FUNCTION "FC_PROG_L1" : VOID
TITLE =FC PROG OVEN LINE 1
{ S7_language := '9(1) Angielski (Stany Zjednoczone)  11.01.2022  09:45:15' }
VERSION : 0.1


VAR_TEMP
  DoorOK : BOOL ;
  ECooling_SP : REAL ;
END_VAR
BEGIN
NETWORK
TITLE =SET FULL PRODUCTION OR REDUCED PRODUCTION MODE
//THIS MODE WILL BE USE AFTER IN SETTING SETPOINTS FOR OVEN FANS (=15FAN01,
//=20FAN01)
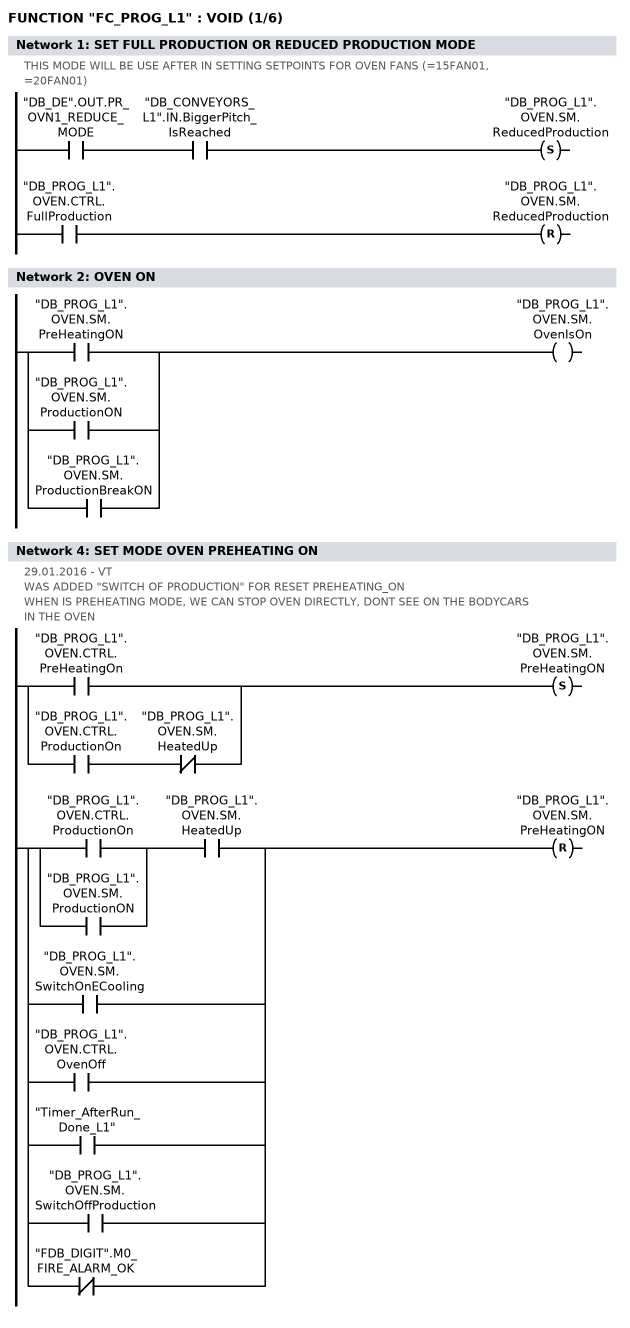
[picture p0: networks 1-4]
      U     "DB_DE".OUT.PR_OVN1_REDUCE_MODE;
      U     "DB_CONVEYORS_L1".IN.BiggerPitch_IsReached;
      S     "DB_PROG_L1".OVEN.SM.ReducedProduction;
      U     "DB_PROG_L1".OVEN.CTRL.FullProduction;
      R     "DB_PROG_L1".OVEN.SM.ReducedProduction;
      NOP   0;
NETWORK
TITLE =OVEN ON

      O     "DB_PROG_L1".OVEN.SM.PreHeatingON;
      O     "DB_PROG_L1".OVEN.SM.ProductionON;
      O     "DB_PROG_L1".OVEN.SM.ProductionBreakON;
      =     "DB_PROG_L1".OVEN.SM.OvenIsOn;
NETWORK
TITLE =SET MODE OF OVEN
//
//************************** SET MODE OF OVEN **********************************
//
NETWORK
TITLE =SET MODE OVEN PREHEATING ON
//29.01.2016 - VT
//WAS ADDED "SWITCH OF PRODUCTION" FOR RESET PREHEATING_ON
//WHEN IS PREHEATING MODE, WE CAN STOP OVEN DIRECTLY, DONT SEE ON THE BODYCARS
//IN THE OVEN
      U(    ;
      O     "DB_PROG_L1".OVEN.CTRL.PreHeatingOn;
      O     ;
      U     "DB_PROG_L1".OVEN.CTRL.ProductionOn;
      UN    "DB_PROG_L1".OVEN.SM.HeatedUp;
      )     ;
      S     "DB_PROG_L1".OVEN.SM.PreHeatingON;
      U(    ;
      U(    ;
      O     "DB_PROG_L1".OVEN.CTRL.ProductionOn;
      O     "DB_PROG_L1".OVEN.SM.ProductionON;
      )     ;
      U     "DB_PROG_L1".OVEN.SM.HeatedUp;
      O     "DB_PROG_L1".OVEN.SM.SwitchOnECooling;
      O     "DB_PROG_L1".OVEN.CTRL.OvenOff;
      O     "Timer_AfterRun_Done_L1";
      O     "DB_PROG_L1".OVEN.SM.SwitchOffProduction;
      ON    "FDB_DIGIT".M0_FIRE_ALARM_OK;
      )     ;
      R     "DB_PROG_L1".OVEN.SM.PreHeatingON;
      NOP   0;
NETWORK
TITLE =SET MODE OVEN PRODUCTION ON
//29.01.2016 - VT
//WAS ADDED ADDITIONAL LOCK FOR RESER PRODUCTION MODE -
//"OVEN_OFF_AFTER_RUN" (M510.0)
//IT MEANS, THAT WE CAN'T STOP OVEN, WHEN WITH BODYCARS INSIDE
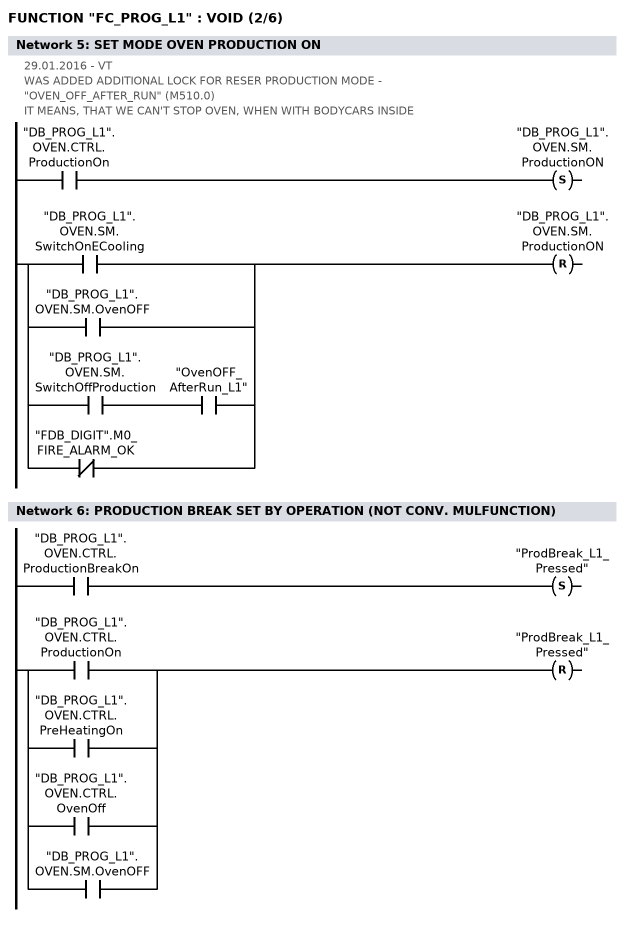
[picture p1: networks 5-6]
      U     "DB_PROG_L1".OVEN.CTRL.ProductionOn;
      S     "DB_PROG_L1".OVEN.SM.ProductionON;
      U(    ;
      O     "DB_PROG_L1".OVEN.SM.SwitchOnECooling;
      O     "DB_PROG_L1".OVEN.SM.OvenOFF;
      O     ;
      U     "DB_PROG_L1".OVEN.SM.SwitchOffProduction;
      U     "OvenOFF_AfterRun_L1";
      ON    "FDB_DIGIT".M0_FIRE_ALARM_OK;
      )     ;
      R     "DB_PROG_L1".OVEN.SM.ProductionON;
      NOP   0;
NETWORK
TITLE =PRODUCTION BREAK SET BY OPERATION (NOT CONV. MULFUNCTION)

      U     "DB_PROG_L1".OVEN.CTRL.ProductionBreakOn;
      S     "ProdBreak_L1_Pressed";
      U(    ;
      O     "DB_PROG_L1".OVEN.CTRL.ProductionOn;
      O     "DB_PROG_L1".OVEN.CTRL.PreHeatingOn;
      O     "DB_PROG_L1".OVEN.CTRL.OvenOff;
      O     "DB_PROG_L1".OVEN.SM.OvenOFF;
      )     ;
      R     "ProdBreak_L1_Pressed";
      NOP   0;
NETWORK
TITLE =SET MODE OVEN PRODUCTION BREAK ON
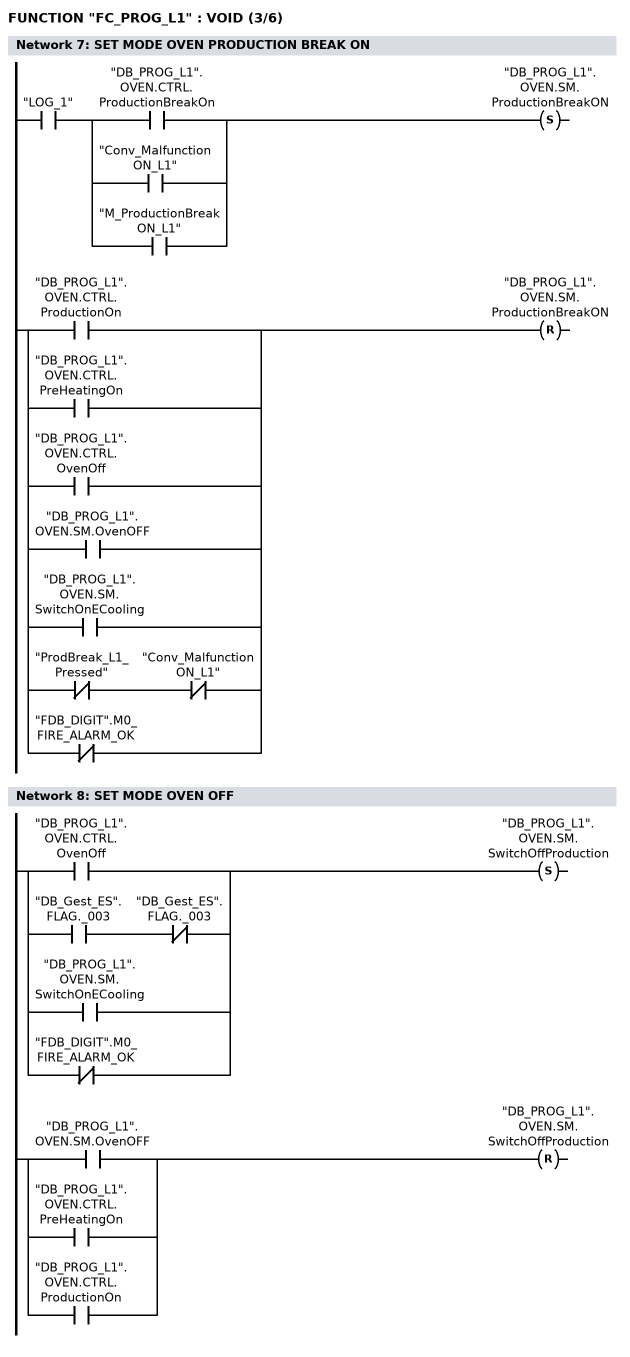
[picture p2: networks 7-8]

      U     "LOG_1";
      U(    ;
      O     "DB_PROG_L1".OVEN.CTRL.ProductionBreakOn;
      O     "Conv_MalfunctionON_L1";
      O     "M_ProductionBreakON_L1";
      )     ;
      S     "DB_PROG_L1".OVEN.SM.ProductionBreakON;
      U(    ;
      O     "DB_PROG_L1".OVEN.CTRL.ProductionOn;
      O     "DB_PROG_L1".OVEN.CTRL.PreHeatingOn;
      O     "DB_PROG_L1".OVEN.CTRL.OvenOff;
      O     "DB_PROG_L1".OVEN.SM.OvenOFF;
      O     "DB_PROG_L1".OVEN.SM.SwitchOnECooling;
      O     ;
      UN    "ProdBreak_L1_Pressed";
      UN    "Conv_MalfunctionON_L1";
      ON    "FDB_DIGIT".M0_FIRE_ALARM_OK;
      )     ;
      R     "DB_PROG_L1".OVEN.SM.ProductionBreakON;
      NOP   0;
NETWORK
TITLE =SET MODE OVEN OFF

      U(    ;
      O     "DB_PROG_L1".OVEN.CTRL.OvenOff;
      O     ;
      U     "DB_Gest_ES".FLAG._003;
      UN    "DB_Gest_ES".FLAG._003;
      O     "DB_PROG_L1".OVEN.SM.SwitchOnECooling;
      ON    "FDB_DIGIT".M0_FIRE_ALARM_OK;
      )     ;
      S     "DB_PROG_L1".OVEN.SM.SwitchOffProduction;
      U(    ;
      O     "DB_PROG_L1".OVEN.SM.OvenOFF;
      O     "DB_PROG_L1".OVEN.CTRL.PreHeatingOn;
      O     "DB_PROG_L1".OVEN.CTRL.ProductionOn;
      )     ;
      R     "DB_PROG_L1".OVEN.SM.SwitchOffProduction;
      NOP   0;
NETWORK
TITLE =AFTER VENTILATION IS FINISHED, OVEN IS OFF
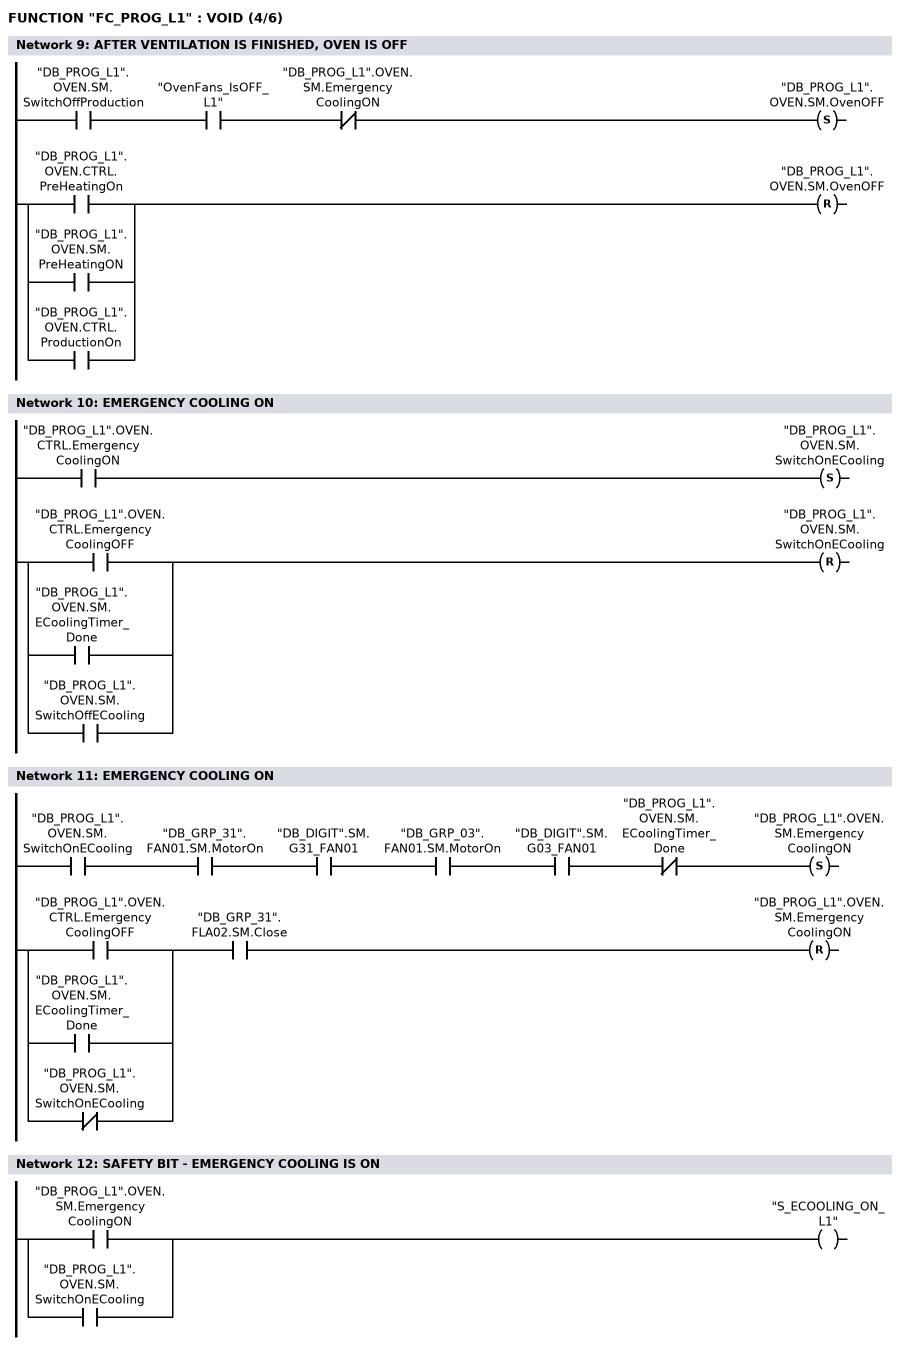
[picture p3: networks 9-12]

      U     "DB_PROG_L1".OVEN.SM.SwitchOffProduction;
      U     "OvenFans_IsOFF_L1";
      UN    "DB_PROG_L1".OVEN.SM.EmergencyCoolingON;
      S     "DB_PROG_L1".OVEN.SM.OvenOFF;
      U(    ;
      O     "DB_PROG_L1".OVEN.CTRL.PreHeatingOn;
      O     "DB_PROG_L1".OVEN.SM.PreHeatingON;
      O     "DB_PROG_L1".OVEN.CTRL.ProductionOn;
      )     ;
      R     "DB_PROG_L1".OVEN.SM.OvenOFF;
      NOP   0;
NETWORK
TITLE =EMERGENCY COOLING ON

      U     "DB_PROG_L1".OVEN.CTRL.EmergencyCoolingON;
      S     "DB_PROG_L1".OVEN.SM.SwitchOnECooling;
      U(    ;
      O     "DB_PROG_L1".OVEN.CTRL.EmergencyCoolingOFF;
      O     "DB_PROG_L1".OVEN.SM.ECoolingTimer_Done;
      O     "DB_PROG_L1".OVEN.SM.SwitchOffECooling;
      )     ;
      R     "DB_PROG_L1".OVEN.SM.SwitchOnECooling;
      NOP   0;
NETWORK
TITLE =EMERGENCY COOLING ON

      U     "DB_PROG_L1".OVEN.SM.SwitchOnECooling;
      U     "DB_GRP_31".FAN01.SM.MotorOn;
      U     "DB_DIGIT".SM.G31_FAN01;
      U     "DB_GRP_03".FAN01.SM.MotorOn;
      U     "DB_DIGIT".SM.G03_FAN01;
      UN    "DB_PROG_L1".OVEN.SM.ECoolingTimer_Done;
      S     "DB_PROG_L1".OVEN.SM.EmergencyCoolingON;
      U(    ;
      O     "DB_PROG_L1".OVEN.CTRL.EmergencyCoolingOFF;
      O     "DB_PROG_L1".OVEN.SM.ECoolingTimer_Done;
      ON    "DB_PROG_L1".OVEN.SM.SwitchOnECooling;
      )     ;
      U     "DB_GRP_31".FLA02.SM.Close;
      R     "DB_PROG_L1".OVEN.SM.EmergencyCoolingON;
      NOP   0;
NETWORK
TITLE =SAFETY BIT - EMERGENCY COOLING IS ON

      O     "DB_PROG_L1".OVEN.SM.EmergencyCoolingON;
      O     "DB_PROG_L1".OVEN.SM.SwitchOnECooling;
      =     "S_ECOOLING_ON_L1";
NETWORK
TITLE =SWITCHING EMERGENCY COOLING OFF
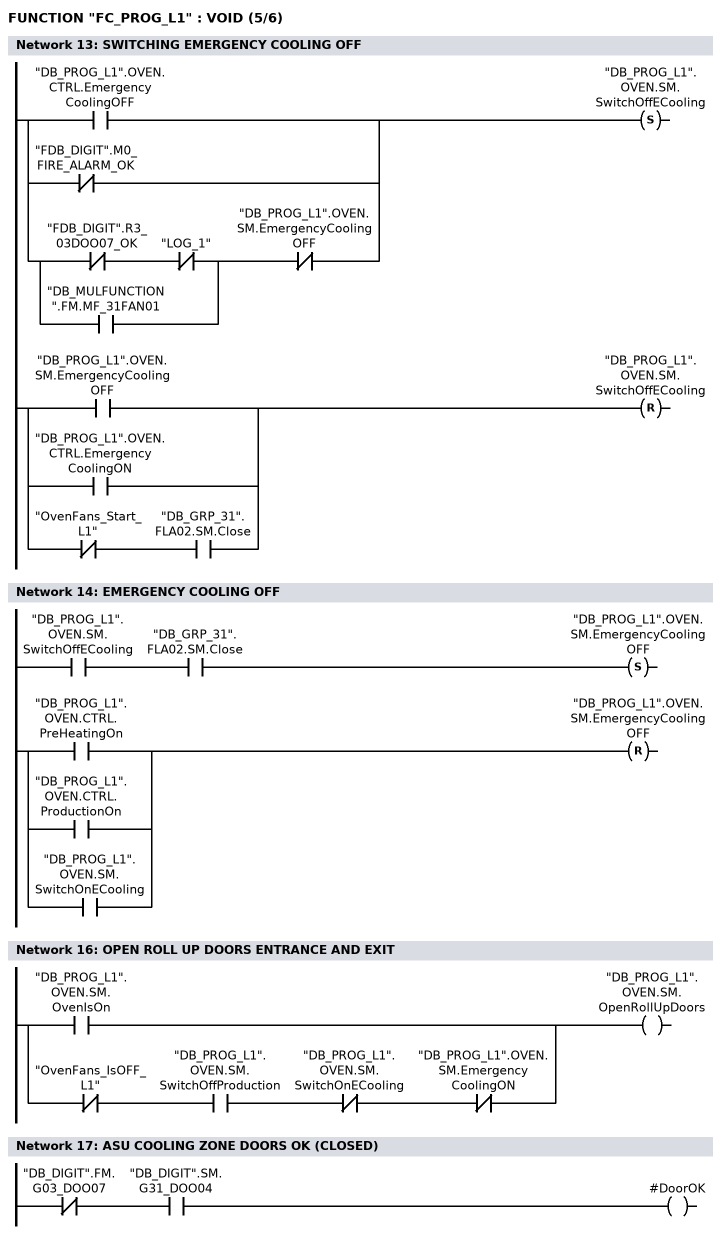
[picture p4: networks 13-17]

      U(    ;
      O     "DB_PROG_L1".OVEN.CTRL.EmergencyCoolingOFF;
      ON    "FDB_DIGIT".M0_FIRE_ALARM_OK;
      O     ;
      U(    ;
      UN    "FDB_DIGIT".R3_03DOO07_OK;
      UN    "LOG_1";
      O     "DB_MULFUNCTION".FM.MF_31FAN01;
      )     ;
      UN    "DB_PROG_L1".OVEN.SM.EmergencyCoolingOFF;
      )     ;
      S     "DB_PROG_L1".OVEN.SM.SwitchOffECooling;
      U(    ;
      O     "DB_PROG_L1".OVEN.SM.EmergencyCoolingOFF;
      O     "DB_PROG_L1".OVEN.CTRL.EmergencyCoolingON;
      O     ;
      UN    "OvenFans_Start_L1";
      U     "DB_GRP_31".FLA02.SM.Close;
      )     ;
      R     "DB_PROG_L1".OVEN.SM.SwitchOffECooling;
      NOP   0;
NETWORK
TITLE =EMERGENCY COOLING OFF

      U     "DB_PROG_L1".OVEN.SM.SwitchOffECooling;
      U     "DB_GRP_31".FLA02.SM.Close;
      S     "DB_PROG_L1".OVEN.SM.EmergencyCoolingOFF;
      U(    ;
      O     "DB_PROG_L1".OVEN.CTRL.PreHeatingOn;
      O     "DB_PROG_L1".OVEN.CTRL.ProductionOn;
      O     "DB_PROG_L1".OVEN.SM.SwitchOnECooling;
      )     ;
      R     "DB_PROG_L1".OVEN.SM.EmergencyCoolingOFF;
      NOP   0;
NETWORK
TITLE =PRE-HEATING MODE
//
//**************************** SET OVEN PRE-HEATING MODE ************************
//
NETWORK
TITLE =OPEN ROLL UP DOORS ENTRANCE AND EXIT

      O     "DB_PROG_L1".OVEN.SM.OvenIsOn;
      O     ;
      UN    "OvenFans_IsOFF_L1";
      U     "DB_PROG_L1".OVEN.SM.SwitchOffProduction;
      UN    "DB_PROG_L1".OVEN.SM.SwitchOnECooling;
      UN    "DB_PROG_L1".OVEN.SM.EmergencyCoolingON;
      =     "DB_PROG_L1".OVEN.SM.OpenRollUpDoors;
NETWORK
TITLE =ASU COOLING ZONE DOORS OK (CLOSED)

      UN    "DB_DIGIT".FM.G03_DOO07;
      U     "DB_DIGIT".SM.G31_DOO04;
      =     #DoorOK;
NETWORK
TITLE =OVEN CHAIN ON
//FROM E-MAIL FROM EN DON'T LOOK ON THE SIGNAL FROM
//CONVEYORS
//"DoorExit_IsMovedFree" - STOP CHAIN IMMEDIATELY AFTER GIVE BACK
//"DoorEntrance_IsMovedFree" AND IS EMERGENCY COOLING ON.
//
//23.04.2016 - VT
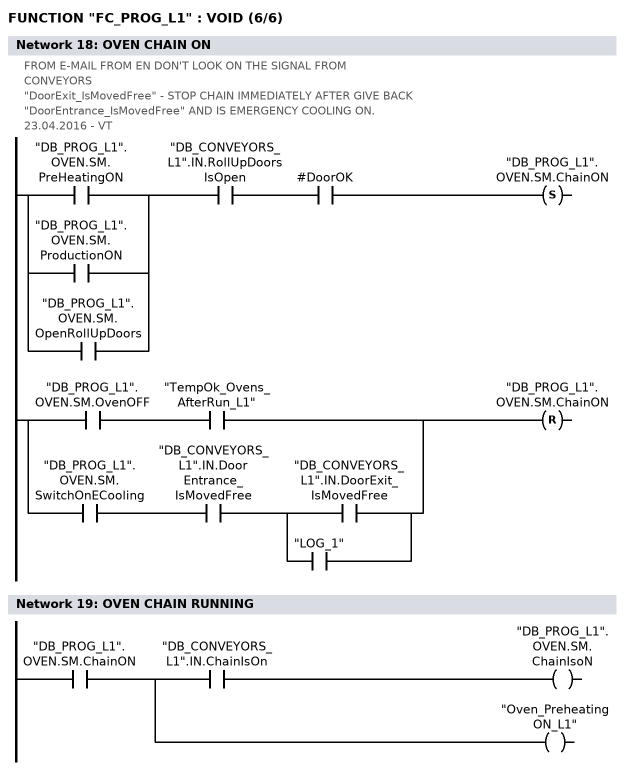
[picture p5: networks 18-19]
      U(    ;
      O     "DB_PROG_L1".OVEN.SM.PreHeatingON;
      O     "DB_PROG_L1".OVEN.SM.ProductionON;
      O     "DB_PROG_L1".OVEN.SM.OpenRollUpDoors;
      )     ;
      U     "DB_CONVEYORS_L1".IN.RollUpDoorsIsOpen;
      U     #DoorOK;
      S     "DB_PROG_L1".OVEN.SM.ChainON;
      U(    ;
      U     "DB_PROG_L1".OVEN.SM.OvenOFF;
      U     "TempOk_Ovens_AfterRun_L1";
      O     ;
      U     "DB_PROG_L1".OVEN.SM.SwitchOnECooling;
      U     "DB_CONVEYORS_L1".IN.DoorEntrance_IsMovedFree;
      U(    ;
      O     "DB_CONVEYORS_L1".IN.DoorExit_IsMovedFree;
      O     "LOG_1";
      )     ;
      )     ;
      R     "DB_PROG_L1".OVEN.SM.ChainON;
      NOP   0;
NETWORK
TITLE =OVEN CHAIN RUNNING

      U     "DB_PROG_L1".OVEN.SM.ChainON;
      =     L      6.0;
      U     L      6.0;
      U     "DB_CONVEYORS_L1".IN.ChainIsOn;
      =     "DB_PROG_L1".OVEN.SM.ChainIsoN;
      U     L      6.0;
      BLD   102;
      =     "Oven_PreheatingON_L1";
NETWORK
TITLE =CLOSE FLAPS =03/=04/=11/=12/=21FLA02 AND OPEN FLAPS =15FLA02/06

      U(    ;
      U     "DB_PROG_L1".OVEN.SM.PreHeatingON;
      S     "CloseFlap_ToMainPos_L1";
      U     "DB_PROG_L1".OVEN.SM.MainPosition;
      R     "CloseFlap_ToMainPos_L1";
      U     "CloseFlap_ToMainPos_L1";
      )     ;
      S     "Open_15FLA06";
      U(    ;
      UN    "DB_PROG_L1".OVEN.SM.OvenIsOn;
      U     "DB_GRP_20".FAN01.SM.MotorOff;
      U     "DB_GRP_15".FAN01.SM.MotorOff;
      L     S5T#30S;
      SE    "T_5_0_1_L1";
      NOP   0;
      NOP   0;
      NOP   0;
      U     "T_5_0_1_L1";
      )     ;
      R     "Open_15FLA06";
      NOP   0;
NETWORK
TITLE =CHECK LIMIT SWITCHES OF =03/=04/=11/=12FLA02
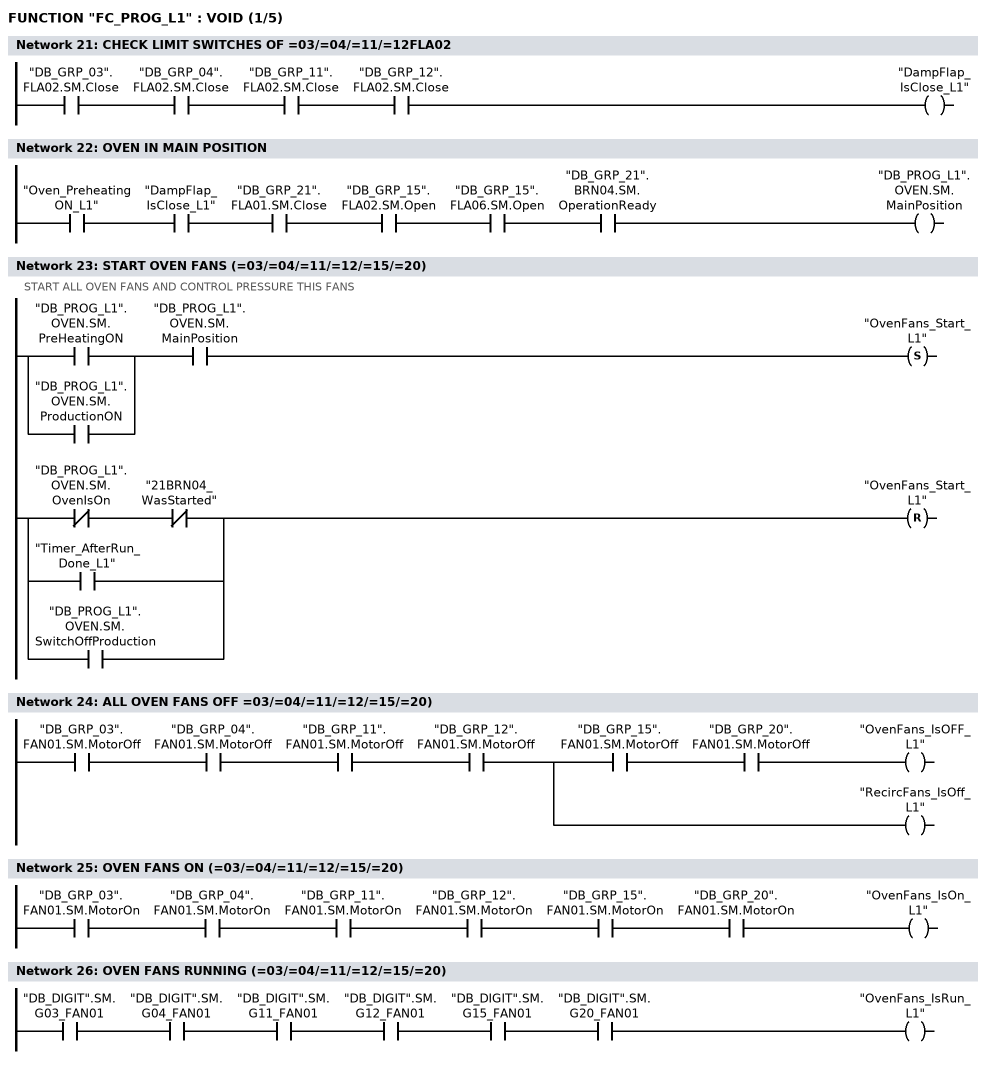
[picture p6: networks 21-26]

      U     "DB_GRP_03".FLA02.SM.Close;
      U     "DB_GRP_04".FLA02.SM.Close;
      U     "DB_GRP_11".FLA02.SM.Close;
      U     "DB_GRP_12".FLA02.SM.Close;
      =     "DampFlap_IsClose_L1";
NETWORK
TITLE =OVEN IN MAIN POSITION

      U     "Oven_PreheatingON_L1";
      U     "DampFlap_IsClose_L1";
      U     "DB_GRP_21".FLA01.SM.Close;
      U     "DB_GRP_15".FLA02.SM.Open;
      U     "DB_GRP_15".FLA06.SM.Open;
      U     "DB_GRP_21".BRN04.SM.OperationReady;
      =     "DB_PROG_L1".OVEN.SM.MainPosition;
NETWORK
TITLE =START OVEN FANS (=03/=04/=11/=12/=15/=20)
//START ALL OVEN FANS AND CONTROL PRESSURE THIS FANS
//
//
      U(    ;
      O     "DB_PROG_L1".OVEN.SM.PreHeatingON;
      O     "DB_PROG_L1".OVEN.SM.ProductionON;
      )     ;
      U     "DB_PROG_L1".OVEN.SM.MainPosition;
      S     "OvenFans_Start_L1";
      U(    ;
      UN    "DB_PROG_L1".OVEN.SM.OvenIsOn;
      UN    "21BRN04_WasStarted";
      O     "Timer_AfterRun_Done_L1";
      O     "DB_PROG_L1".OVEN.SM.SwitchOffProduction;
      )     ;
      R     "OvenFans_Start_L1";
      NOP   0;
NETWORK
TITLE =ALL OVEN FANS OFF =03/=04/=11/=12/=15/=20)

      U     "DB_GRP_03".FAN01.SM.MotorOff;
      U     "DB_GRP_04".FAN01.SM.MotorOff;
      U     "DB_GRP_11".FAN01.SM.MotorOff;
      U     "DB_GRP_12".FAN01.SM.MotorOff;
      =     L      6.0;
      U     L      6.0;
      U     "DB_GRP_15".FAN01.SM.MotorOff;
      U     "DB_GRP_20".FAN01.SM.MotorOff;
      =     "OvenFans_IsOFF_L1";
      U     L      6.0;
      BLD   102;
      =     "RecircFans_IsOff_L1";
NETWORK
TITLE =OVEN FANS ON (=03/=04/=11/=12/=15/=20)

      U     "DB_GRP_03".FAN01.SM.MotorOn;
      U     "DB_GRP_04".FAN01.SM.MotorOn;
      U     "DB_GRP_11".FAN01.SM.MotorOn;
      U     "DB_GRP_12".FAN01.SM.MotorOn;
      U     "DB_GRP_15".FAN01.SM.MotorOn;
      U     "DB_GRP_20".FAN01.SM.MotorOn;
      =     "OvenFans_IsOn_L1";
NETWORK
TITLE =OVEN FANS RUNNING (=03/=04/=11/=12/=15/=20)

      U     "DB_DIGIT".SM.G03_FAN01;
      U     "DB_DIGIT".SM.G04_FAN01;
      U     "DB_DIGIT".SM.G11_FAN01;
      U     "DB_DIGIT".SM.G12_FAN01;
      U     "DB_DIGIT".SM.G15_FAN01;
      U     "DB_DIGIT".SM.G20_FAN01;
      =     "OvenFans_IsRun_L1";
NETWORK
TITLE =PRE-PURGING TIMER
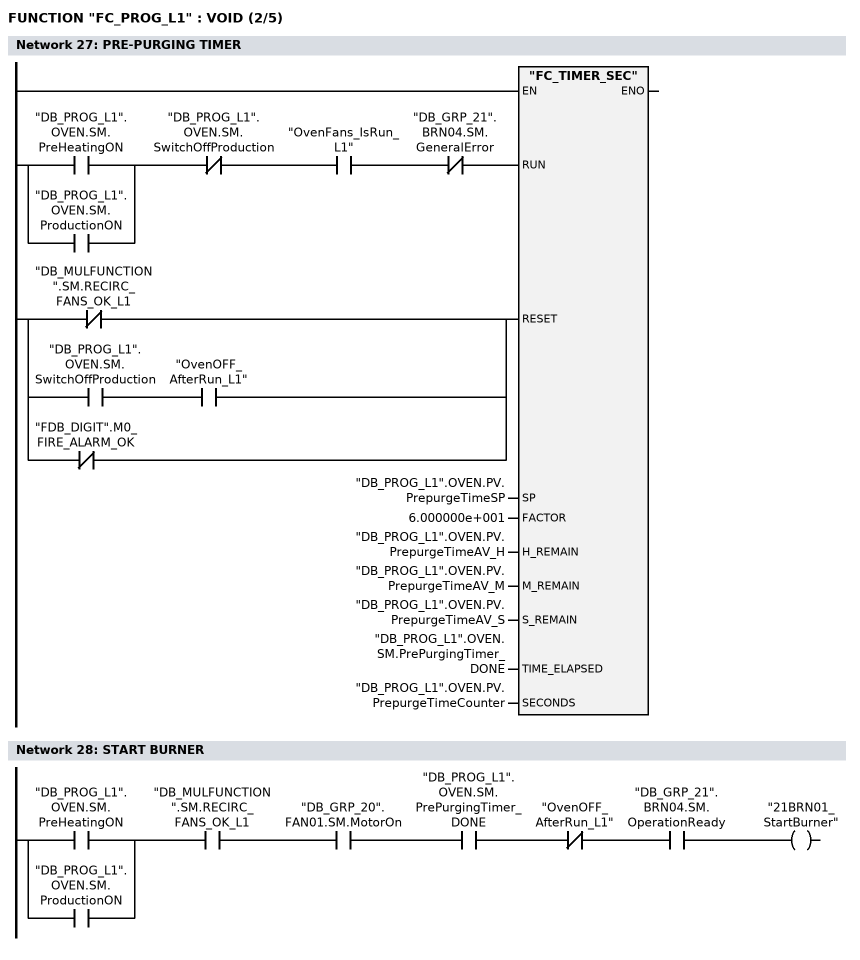
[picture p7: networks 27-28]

      U(    ;
      O     "DB_PROG_L1".OVEN.SM.PreHeatingON;
      O     "DB_PROG_L1".OVEN.SM.ProductionON;
      )     ;
      UN    "DB_PROG_L1".OVEN.SM.SwitchOffProduction;
      U     "OvenFans_IsRun_L1";
      UN    "DB_GRP_21".BRN04.SM.GeneralError;
      =     L      6.0;
      BLD   103;
      U(    ;
      ON    "DB_MULFUNCTION".SM.RECIRC_FANS_OK_L1;
      O     ;
      U     "DB_PROG_L1".OVEN.SM.SwitchOffProduction;
      U     "OvenOFF_AfterRun_L1";
      ON    "FDB_DIGIT".M0_FIRE_ALARM_OK;
      )     ;
      =     L      6.1;
      BLD   103;
      CALL "FC_TIMER_SEC" (
           RUN                      := L      6.0,
           RESET                    := L      6.1,
           SP                       := "DB_PROG_L1".OVEN.PV.PrepurgeTimeSP,
           FACTOR                   := 6.000000e+001,
           H_REMAIN                 := "DB_PROG_L1".OVEN.PV.PrepurgeTimeAV_H,
           M_REMAIN                 := "DB_PROG_L1".OVEN.PV.PrepurgeTimeAV_M,
           S_REMAIN                 := "DB_PROG_L1".OVEN.PV.PrepurgeTimeAV_S,
           TIME_ELAPSED             := "DB_PROG_L1".OVEN.SM.PrePurgingTimer_DONE,
           SECONDS                  := "DB_PROG_L1".OVEN.PV.PrepurgeTimeCounter);
      NOP   0;
NETWORK
TITLE =START BURNER

      U(    ;
      O     "DB_PROG_L1".OVEN.SM.PreHeatingON;
      O     "DB_PROG_L1".OVEN.SM.ProductionON;
      )     ;
      U     "DB_MULFUNCTION".SM.RECIRC_FANS_OK_L1;
      U     "DB_GRP_20".FAN01.SM.MotorOn;
      U     "DB_PROG_L1".OVEN.SM.PrePurgingTimer_DONE;
      UN    "OvenOFF_AfterRun_L1";
      U     "DB_GRP_21".BRN04.SM.OperationReady;
      =     "21BRN01_StartBurner";
NETWORK
TITLE =OVEN GROUP =03/=04/=11/=12/=15 TEMPERATURE OK
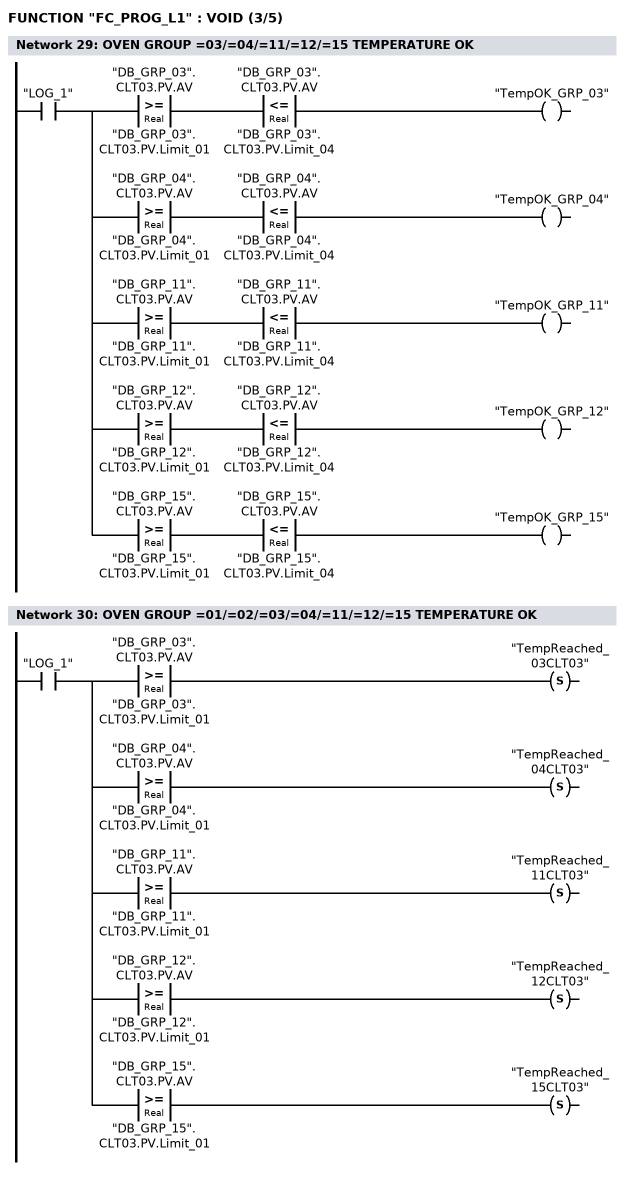
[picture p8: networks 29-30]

      U     "LOG_1";
      =     L      6.0;
      U     L      6.0;
      U(    ;
      L     "DB_GRP_03".CLT03.PV.AV;
      L     "DB_GRP_03".CLT03.PV.Limit_01;
      >=R   ;
      )     ;
      U(    ;
      L     "DB_GRP_03".CLT03.PV.AV;
      L     "DB_GRP_03".CLT03.PV.Limit_04;
      <=R   ;
      )     ;
      =     "TempOK_GRP_03";
      U     L      6.0;
      U(    ;
      L     "DB_GRP_04".CLT03.PV.AV;
      L     "DB_GRP_04".CLT03.PV.Limit_01;
      >=R   ;
      )     ;
      U(    ;
      L     "DB_GRP_04".CLT03.PV.AV;
      L     "DB_GRP_04".CLT03.PV.Limit_04;
      <=R   ;
      )     ;
      =     "TempOK_GRP_04";
      U     L      6.0;
      U(    ;
      L     "DB_GRP_11".CLT03.PV.AV;
      L     "DB_GRP_11".CLT03.PV.Limit_01;
      >=R   ;
      )     ;
      U(    ;
      L     "DB_GRP_11".CLT03.PV.AV;
      L     "DB_GRP_11".CLT03.PV.Limit_04;
      <=R   ;
      )     ;
      =     "TempOK_GRP_11";
      U     L      6.0;
      U(    ;
      L     "DB_GRP_12".CLT03.PV.AV;
      L     "DB_GRP_12".CLT03.PV.Limit_01;
      >=R   ;
      )     ;
      U(    ;
      L     "DB_GRP_12".CLT03.PV.AV;
      L     "DB_GRP_12".CLT03.PV.Limit_04;
      <=R   ;
      )     ;
      =     "TempOK_GRP_12";
      U     L      6.0;
      U(    ;
      L     "DB_GRP_15".CLT03.PV.AV;
      L     "DB_GRP_15".CLT03.PV.Limit_01;
      >=R   ;
      )     ;
      U(    ;
      L     "DB_GRP_15".CLT03.PV.AV;
      L     "DB_GRP_15".CLT03.PV.Limit_04;
      <=R   ;
      )     ;
      =     "TempOK_GRP_15";
NETWORK
TITLE =OVEN GROUP =01/=02/=03/=04/=11/=12/=15 TEMPERATURE OK

      U     "LOG_1";
      =     L      6.0;
      U     L      6.0;
      U(    ;
      L     "DB_GRP_03".CLT03.PV.AV;
      L     "DB_GRP_03".CLT03.PV.Limit_01;
      >=R   ;
      )     ;
      S     "TempReached_03CLT03";
      U     L      6.0;
      U(    ;
      L     "DB_GRP_04".CLT03.PV.AV;
      L     "DB_GRP_04".CLT03.PV.Limit_01;
      >=R   ;
      )     ;
      S     "TempReached_04CLT03";
      U     L      6.0;
      U(    ;
      L     "DB_GRP_11".CLT03.PV.AV;
      L     "DB_GRP_11".CLT03.PV.Limit_01;
      >=R   ;
      )     ;
      S     "TempReached_11CLT03";
      U     L      6.0;
      U(    ;
      L     "DB_GRP_12".CLT03.PV.AV;
      L     "DB_GRP_12".CLT03.PV.Limit_01;
      >=R   ;
      )     ;
      S     "TempReached_12CLT03";
      U     L      6.0;
      U(    ;
      L     "DB_GRP_15".CLT03.PV.AV;
      L     "DB_GRP_15".CLT03.PV.Limit_01;
      >=R   ;
      )     ;
      S     "TempReached_15CLT03";
NETWORK
TITLE =TEMPERATAURE OK
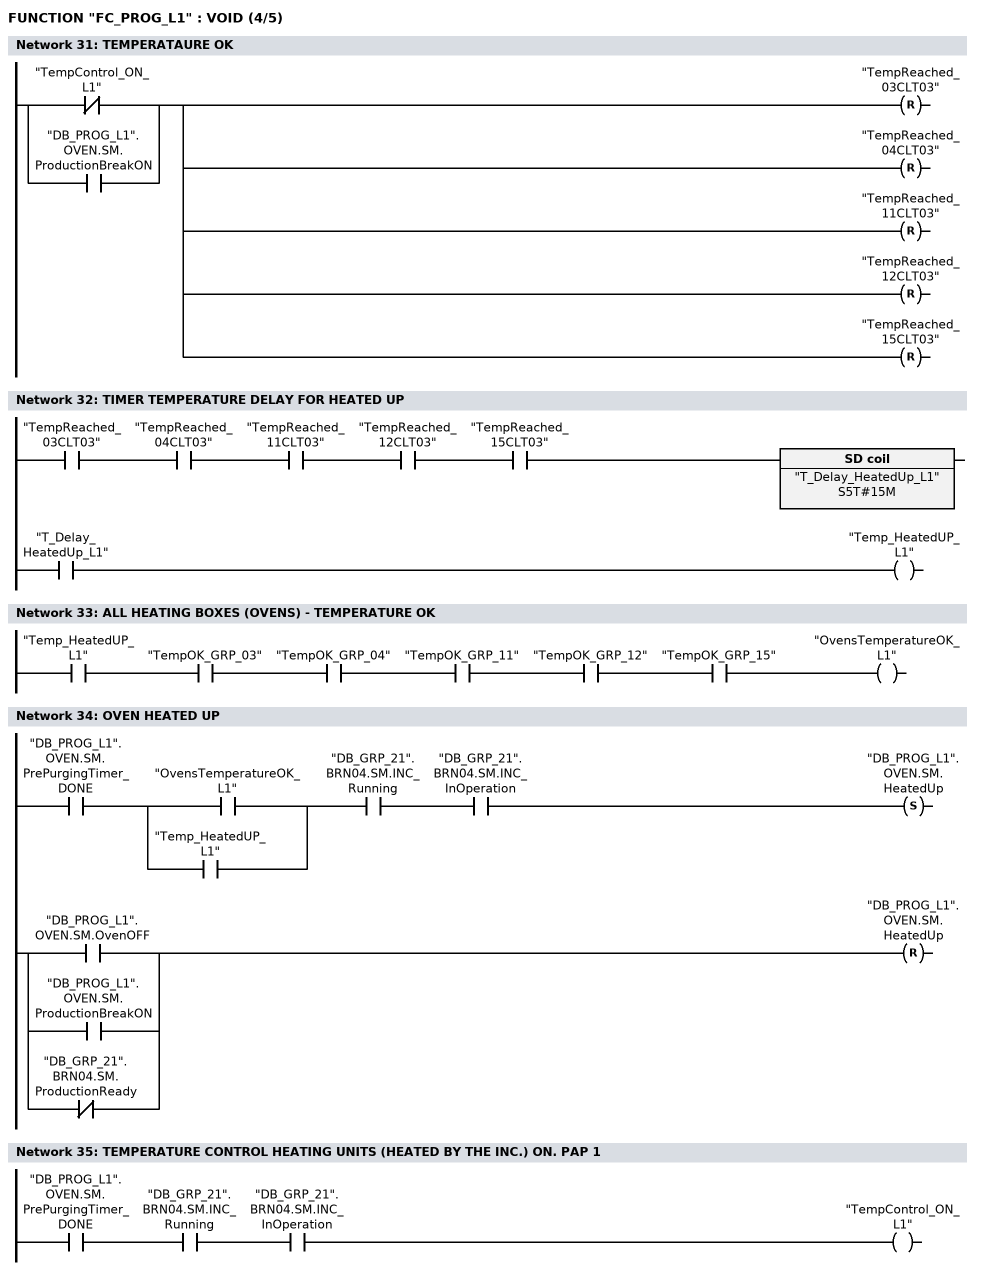
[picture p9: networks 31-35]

      ON    "TempControl_ON_L1";
      O     "DB_PROG_L1".OVEN.SM.ProductionBreakON;
      R     "TempReached_03CLT03";
      R     "TempReached_04CLT03";
      R     "TempReached_11CLT03";
      R     "TempReached_12CLT03";
      R     "TempReached_15CLT03";
NETWORK
TITLE =TIMER TEMPERATURE DELAY FOR HEATED UP

      U     "TempReached_03CLT03";
      U     "TempReached_04CLT03";
      U     "TempReached_11CLT03";
      U     "TempReached_12CLT03";
      U     "TempReached_15CLT03";
      L     S5T#15M;
      SE    "T_Delay_HeatedUp_L1";
      NOP   0;
      NOP   0;
      NOP   0;
      U     "T_Delay_HeatedUp_L1";
      =     "Temp_HeatedUP_L1";
NETWORK
TITLE =ALL HEATING BOXES (OVENS) - TEMPERATURE OK

      U     "Temp_HeatedUP_L1";
      U     "TempOK_GRP_03";
      U     "TempOK_GRP_04";
      U     "TempOK_GRP_11";
      U     "TempOK_GRP_12";
      U     "TempOK_GRP_15";
      =     "OvensTemperatureOK_L1";
NETWORK
TITLE =OVEN HEATED UP

      U     "DB_PROG_L1".OVEN.SM.PrePurgingTimer_DONE;
      U(    ;
      O     "OvensTemperatureOK_L1";
      O     "Temp_HeatedUP_L1";
      )     ;
      U     "DB_GRP_21".BRN04.SM.INC_Running;
      U     "DB_GRP_21".BRN04.SM.INC_InOperation;
      S     "DB_PROG_L1".OVEN.SM.HeatedUp;
      U(    ;
      O     "DB_PROG_L1".OVEN.SM.OvenOFF;
      O     "DB_PROG_L1".OVEN.SM.ProductionBreakON;
      ON    "DB_GRP_21".BRN04.SM.ProductionReady;
      )     ;
      R     "DB_PROG_L1".OVEN.SM.HeatedUp;
      NOP   0;
NETWORK
TITLE =TEMPERATURE CONTROL HEATING UNITS (HEATED BY THE INC.) ON. PAP 1

      U     "DB_PROG_L1".OVEN.SM.PrePurgingTimer_DONE;
      U     "DB_GRP_21".BRN04.SM.INC_Running;
      U     "DB_GRP_21".BRN04.SM.INC_InOperation;
      =     "TempControl_ON_L1";
NETWORK
TITLE =BURNER =21BRN04 WAS STARTED
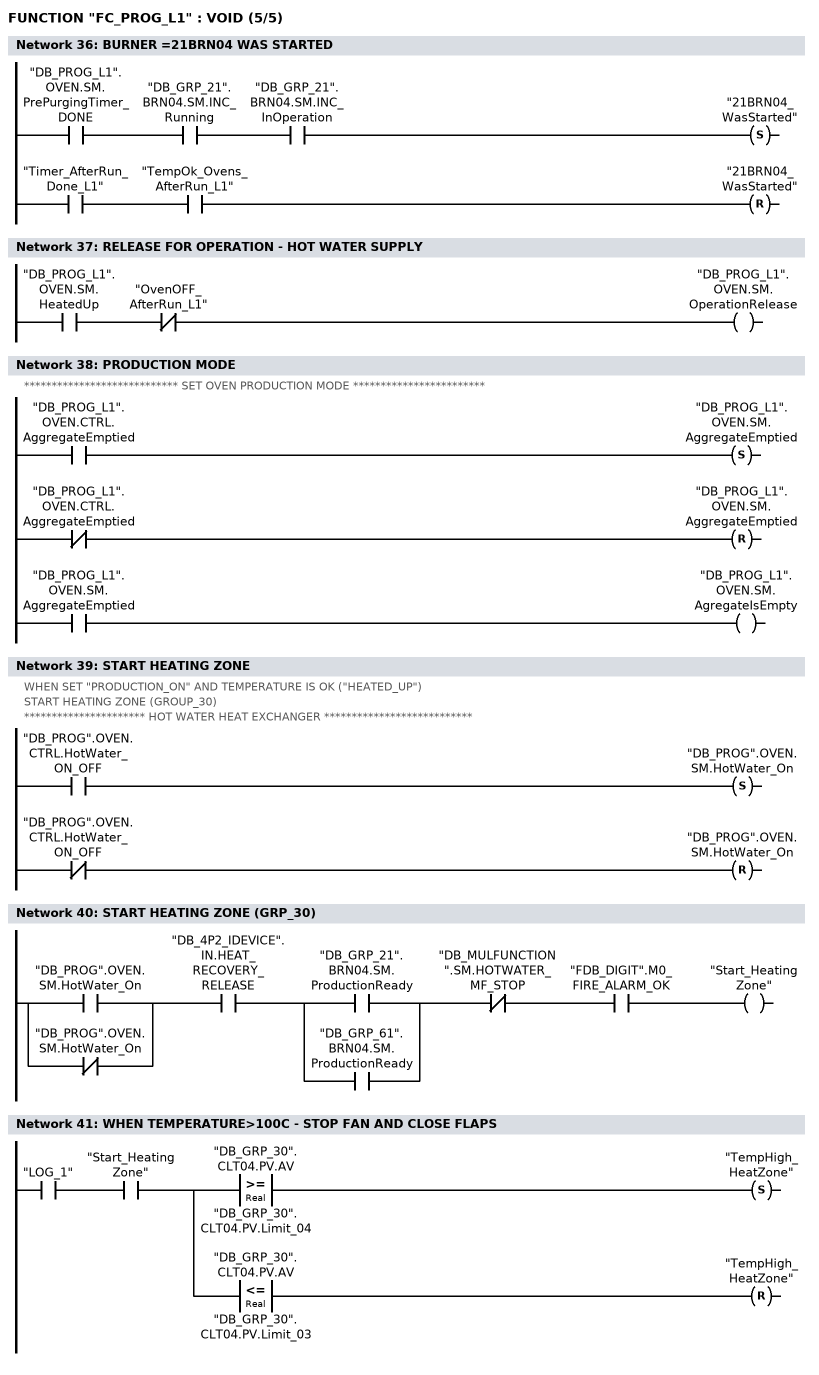
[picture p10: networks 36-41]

      U     "DB_PROG_L1".OVEN.SM.PrePurgingTimer_DONE;
      U     "DB_GRP_21".BRN04.SM.INC_Running;
      U     "DB_GRP_21".BRN04.SM.INC_InOperation;
      S     "21BRN04_WasStarted";
      U     "Timer_AfterRun_Done_L1";
      U     "TempOk_Ovens_AfterRun_L1";
      R     "21BRN04_WasStarted";
      NOP   0;
NETWORK
TITLE =RELEASE FOR OPERATION - HOT WATER SUPPLY

      U     "DB_PROG_L1".OVEN.SM.HeatedUp;
      UN    "OvenOFF_AfterRun_L1";
      =     "DB_PROG_L1".OVEN.SM.OperationRelease;
NETWORK
TITLE =PRODUCTION MODE
//
//**************************** SET OVEN PRODUCTION MODE ************************
//
      U     "DB_PROG_L1".OVEN.CTRL.AggregateEmptied;
      S     "DB_PROG_L1".OVEN.SM.AggregateEmptied;
      UN    "DB_PROG_L1".OVEN.CTRL.AggregateEmptied;
      R     "DB_PROG_L1".OVEN.SM.AggregateEmptied;
      U     "DB_PROG_L1".OVEN.SM.AggregateEmptied;
      =     "DB_PROG_L1".OVEN.SM.AgregateIsEmpty;
NETWORK
TITLE =START HEATING ZONE
//WHEN SET "PRODUCTION_ON" AND TEMPERATURE IS OK ("HEATED_UP")
//START HEATING ZONE (GROUP_30)
//
//********************** HOT WATER HEAT EXCHANGER ***************************
//
      U     "DB_PROG".OVEN.CTRL.HotWater_ON_OFF;
      S     "DB_PROG".OVEN.SM.HotWater_On;
      UN    "DB_PROG".OVEN.CTRL.HotWater_ON_OFF;
      R     "DB_PROG".OVEN.SM.HotWater_On;
      NOP   0;
NETWORK
TITLE =START HEATING ZONE (GRP_30)

      U(    ;
      O     "DB_PROG".OVEN.SM.HotWater_On;
      ON    "DB_PROG".OVEN.SM.HotWater_On;
      )     ;
      U     "DB_4P2_IDEVICE".IN.HEAT_RECOVERY_RELEASE;
      U(    ;
      O     "DB_GRP_21".BRN04.SM.ProductionReady;
      O     "DB_GRP_61".BRN04.SM.ProductionReady;
      )     ;
      UN    "DB_MULFUNCTION".SM.HOTWATER_MF_STOP;
      U     "FDB_DIGIT".M0_FIRE_ALARM_OK;
      =     "Start_HeatingZone";
NETWORK
TITLE =WHEN TEMPERATURE>100C - STOP FAN AND CLOSE FLAPS

      U     "LOG_1";
      U     "Start_HeatingZone";
      =     L      6.0;
      U     L      6.0;
      U(    ;
      L     "DB_GRP_30".CLT04.PV.AV;
      L     "DB_GRP_30".CLT04.PV.Limit_04;
      >=R   ;
      )     ;
      S     "TempHigh_HeatZone";
      U     L      6.0;
      U(    ;
      L     "DB_GRP_30".CLT04.PV.AV;
      L     "DB_GRP_30".CLT04.PV.Limit_03;
      <=R   ;
      )     ;
      R     "TempHigh_HeatZone";
NETWORK
TITLE =OPEN FLAPS =30VA11, =30FLA02, =30FLA03 IN HEATING ZONE

      U(    ;
      U     "Start_HeatingZone";
      U     "DB_GRP_30".VA11.SM.Open;
      U     "DB_DIGIT".SM.G30_MR05S1;
      U     "DB_DIGIT".SM.G30_MR05S2;
      L     S5T#30S;
      SE    "T_OpenFlap_HotWater";
      NOP   0;
      NOP   0;
      NOP   0;
      U     "T_OpenFlap_HotWater";
      )     ;
      S     "OpenFlap_HeatZone";
      U(    ;
      ON    "Start_HeatingZone";
      ON    "DB_GRP_30".VA11.SM.Open;
      ON    "DB_GRP_30".PP10.SM.MotorOn;
      O     "TempHigh_HeatZone";
      )     ;
      U     "DB_GRP_30".FAN01.SM.MotorOff;
      R     "OpenFlap_HeatZone";
      NOP   0;
NETWORK
TITLE =START FAN HEAT EXCHANGER =30FAN01
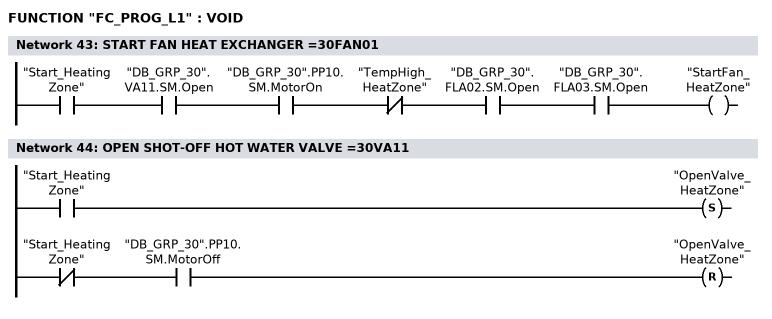
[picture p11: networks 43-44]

      U     "Start_HeatingZone";
      U     "DB_GRP_30".VA11.SM.Open;
      U     "DB_GRP_30".PP10.SM.MotorOn;
      UN    "TempHigh_HeatZone";
      U     "DB_GRP_30".FLA02.SM.Open;
      U     "DB_GRP_30".FLA03.SM.Open;
      =     "StartFan_HeatZone";
NETWORK
TITLE =OPEN SHOT-OFF HOT WATER VALVE =30VA11

      U     "Start_HeatingZone";
      S     "OpenValve_HeatZone";
      UN    "Start_HeatingZone";
      U     "DB_GRP_30".PP10.SM.MotorOff;
      R     "OpenValve_HeatZone";
      NOP   0;
NETWORK
TITLE =START HOT WATER PUMP =30PP10 IN HEATING ZONE

      U     "Start_HeatingZone";
      U     "DB_GRP_30".VA11.SM.Open;
      S     "StartPump_HeatZone";
      U(    ;
      O(    ;
      UN    "Start_HeatingZone";
      L     S5T#20S;
      SE    "Timer_PumpOFF";
      NOP   0;
      NOP   0;
      NOP   0;
      U     "Timer_PumpOFF";
      )     ;
      ON    "DB_GRP_30".VA11.SM.Open;
      )     ;
      R     "StartPump_HeatZone";
      NOP   0;
NETWORK
TITLE =START COOLING ZONE
//WHEN SET "PRODUCTION_ON" AND TEMPERATURE IS OK ("HEATED_UP")
//START COOLING ZONE (GROUP_31)
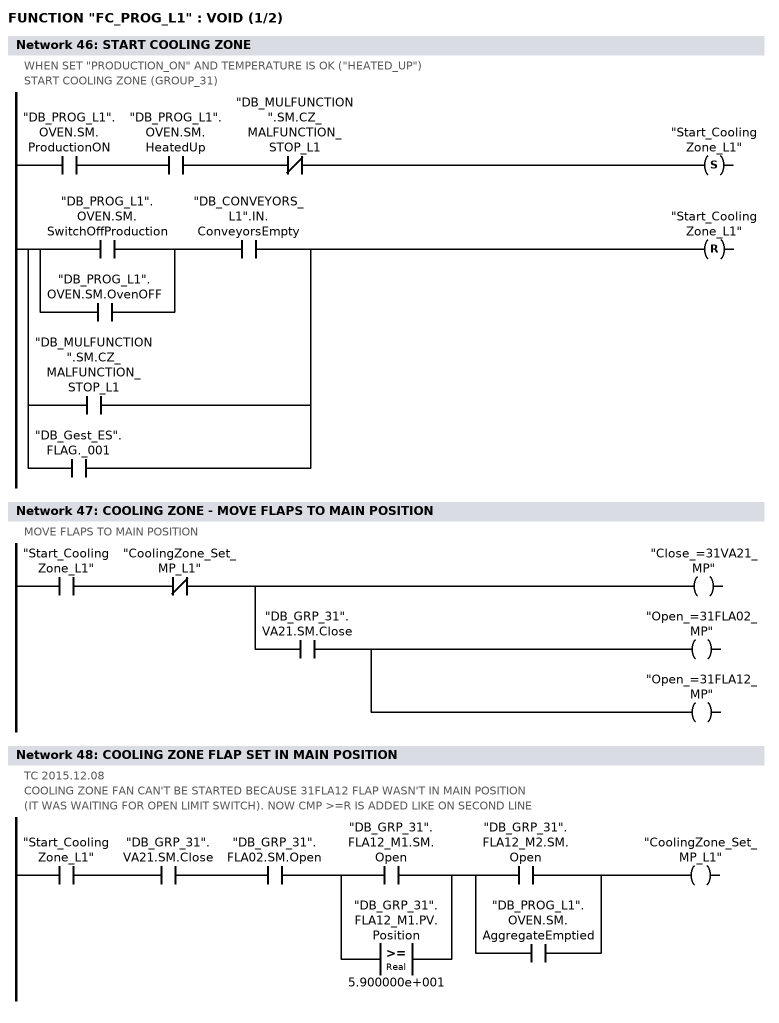
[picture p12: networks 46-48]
      U     "DB_PROG_L1".OVEN.SM.ProductionON;
      U     "DB_PROG_L1".OVEN.SM.HeatedUp;
      UN    "DB_MULFUNCTION".SM.CZ_MALFUNCTION_STOP_L1;
      S     "Start_CoolingZone_L1";
      U(    ;
      U(    ;
      O     "DB_PROG_L1".OVEN.SM.SwitchOffProduction;
      O     "DB_PROG_L1".OVEN.SM.OvenOFF;
      )     ;
      U     "DB_CONVEYORS_L1".IN.ConveyorsEmpty;
      O     "DB_MULFUNCTION".SM.CZ_MALFUNCTION_STOP_L1;
      O     "DB_Gest_ES".FLAG._001;
      )     ;
      R     "Start_CoolingZone_L1";
      NOP   0;
NETWORK
TITLE =COOLING ZONE - MOVE FLAPS TO MAIN POSITION
//MOVE FLAPS TO MAIN POSITION
      U     "Start_CoolingZone_L1";
      UN    "CoolingZone_Set_MP_L1";
      =     L      6.0;
      U     L      6.0;
      BLD   102;
      =     "Close_=31VA21_MP";
      U     L      6.0;
      U     "DB_GRP_31".VA21.SM.Close;
      =     "Open_=31FLA02_MP";
      =     "Open_=31FLA12_MP";
NETWORK
TITLE =COOLING ZONE FLAP SET IN MAIN POSITION
//TC 2015.12.08
//
//COOLING ZONE FAN CAN'T BE STARTED BECAUSE 31FLA12 FLAP WASN'T IN MAIN POSITION
//(IT WAS WAITING FOR OPEN LIMIT SWITCH). NOW CMP >=R IS ADDED LIKE ON SECOND LINE
//
      U     "Start_CoolingZone_L1";
      U     "DB_GRP_31".VA21.SM.Close;
      U     "DB_GRP_31".FLA02.SM.Open;
      U(    ;
      O     "DB_GRP_31".FLA12_M1.SM.Open;
      O(    ;
      L     "DB_GRP_31".FLA12_M1.PV.Position;
      L     5.900000e+001;
      >=R   ;
      )     ;
      )     ;
      U(    ;
      O     "DB_GRP_31".FLA12_M2.SM.Open;
      O     "DB_PROG_L1".OVEN.SM.AggregateEmptied;
      )     ;
      =     "CoolingZone_Set_MP_L1";
NETWORK
TITLE =START FANS OF COOLING ZONE
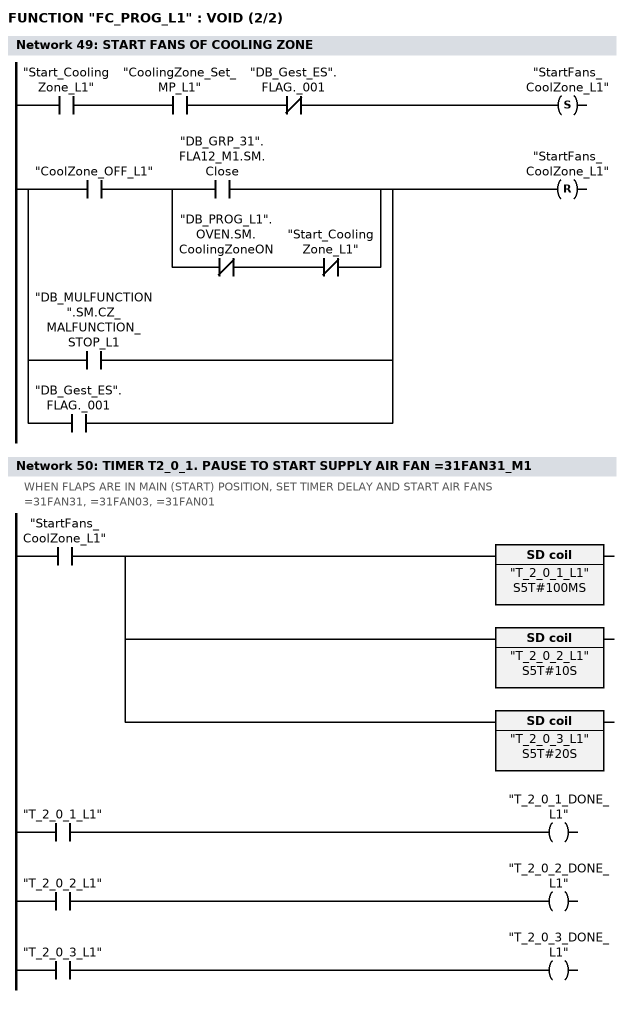
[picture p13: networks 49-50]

      U     "Start_CoolingZone_L1";
      U     "CoolingZone_Set_MP_L1";
      UN    "DB_Gest_ES".FLAG._001;
      S     "StartFans_CoolZone_L1";
      U(    ;
      U     "CoolZone_OFF_L1";
      U(    ;
      O     "DB_GRP_31".FLA12_M1.SM.Close;
      O     ;
      UN    "DB_PROG_L1".OVEN.SM.CoolingZoneON;
      UN    "Start_CoolingZone_L1";
      )     ;
      O     "DB_MULFUNCTION".SM.CZ_MALFUNCTION_STOP_L1;
      O     "DB_Gest_ES".FLAG._001;
      )     ;
      R     "StartFans_CoolZone_L1";
      NOP   0;
NETWORK
TITLE =TIMER T2_0_1. PAUSE TO START SUPPLY AIR FAN =31FAN31_M1
//WHEN FLAPS ARE IN MAIN (START) POSITION, SET TIMER DELAY AND START AIR FANS
//=31FAN31, =31FAN03, =31FAN01
      U     "StartFans_CoolZone_L1";
      =     L      6.0;
      U     L      6.0;
      L     S5T#100MS;
      SE    "T_2_0_1_L1";
      NOP   0;
      NOP   0;
      NOP   0;
      U     "T_2_0_1_L1";
      =     "T_2_0_1_DONE_L1";
      U     L      6.0;
      L     S5T#10S;
      SE    "T_2_0_2_L1";
      NOP   0;
      NOP   0;
      NOP   0;
      U     "T_2_0_2_L1";
      =     "T_2_0_2_DONE_L1";
      U     L      6.0;
      L     S5T#20S;
      SE    "T_2_0_3_L1";
      NOP   0;
      NOP   0;
      NOP   0;
      U     "T_2_0_3_L1";
      =     "T_2_0_3_DONE_L1";
NETWORK
TITLE =WHEN ALL FANS RUNNING AND PRESSURE SENSORS ARE OK
//WHEN TEMPERATURE IN ALL HEATING BOXES OK, FANS RUNNING AND PRESSURE SENSORS ARE
//OK - SET STATUS "RELEASE OF PRODUCTION OVEN" AND "RELEASE FOR CONVEYING"
      U(    ;
      U(    ;
      U     "DB_GRP_31".FAN01.SM.MotorOn;
      U     "DB_DIGIT".SM.G31_FAN01;
      U     "DB_GRP_31".FAN03.SM.MotorOn;
      U     "DB_DIGIT".SM.G31_FAN03;
      U     "DB_GRP_31".FAN31.SM.MotorOn;
      U     "DB_DIGIT".SM.G31_FAN31;
      O     "DB_Gest_ES".FLAG._013;
      O     "DB_Gest_ES".FLAG._001;
      )     ;
      U     "OvensTemperatureOK_L1";
      L     S5T#1M;
      SA    "CONV_LINE1_PROD_REL_DEL";
      NOP   0;
      NOP   0;
      NOP   0;
      U     "CONV_LINE1_PROD_REL_DEL";
      )     ;
      U     "DB_MULFUNCTION".SM.RECIRC_FANS_OK_L1;
      U     "OvenFans_IsRun_L1";
      U     "OvenFans_IsOn_L1";
      U     "DB_PROG_L1".OVEN.SM.ProductionON;
      UN    "DB_PROG_L1".OVEN.SM.ProductionBreakON;
      UN    "DB_PROG_L1".OVEN.SM.SwitchOffProduction;
      UN    "DB_PROG_L1".OVEN.SM.EmergencyCoolingON;
      =     "DB_PROG_L1".OVEN.SM.ProductionRelease;
NETWORK
TITLE =COOLING ZONE ON
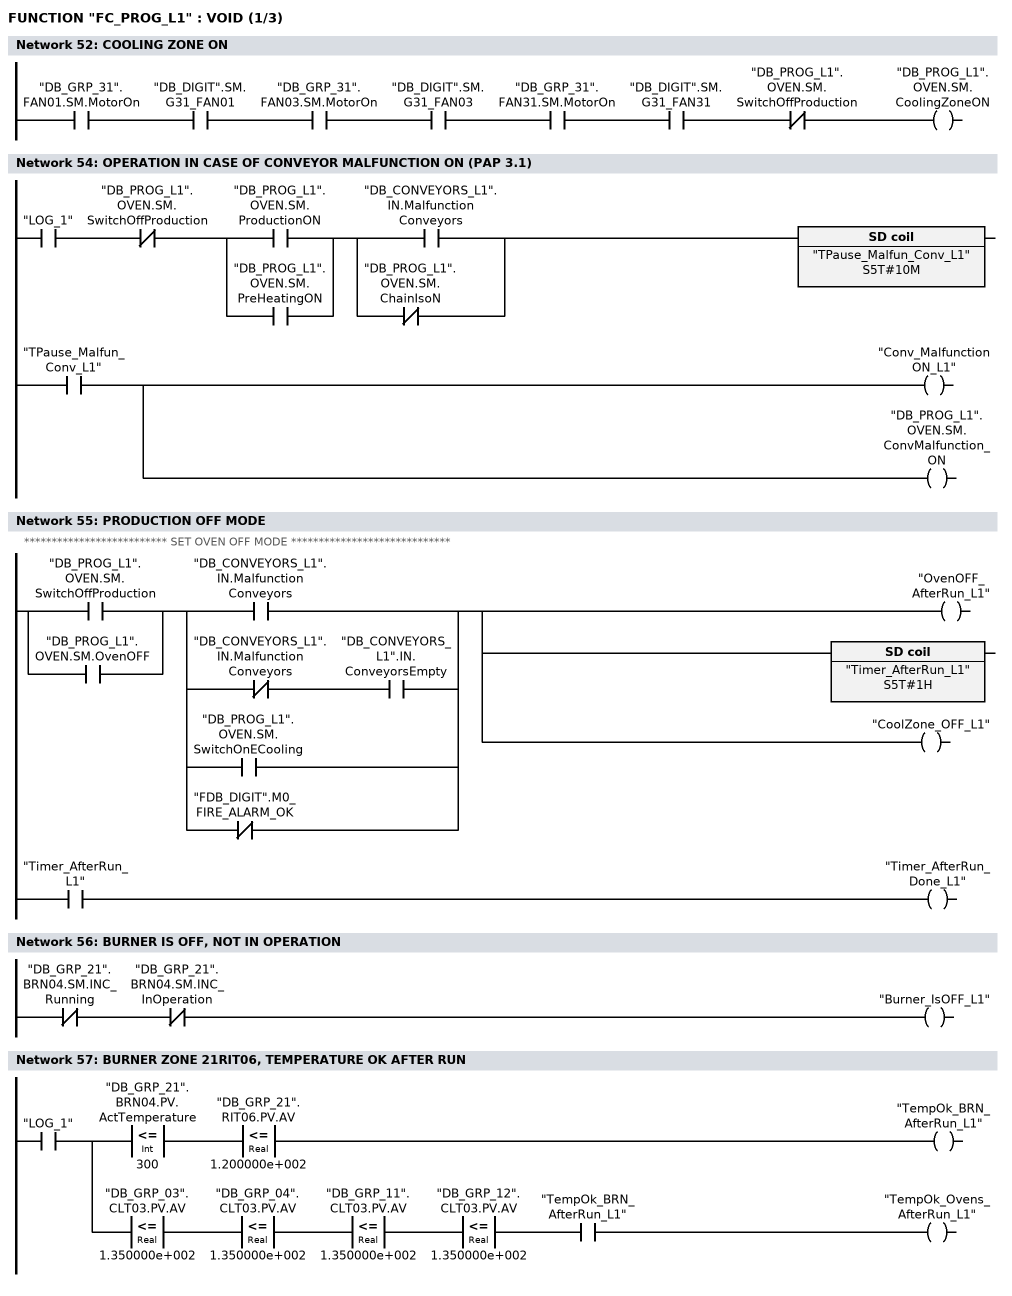
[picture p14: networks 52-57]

      U     "DB_GRP_31".FAN01.SM.MotorOn;
      U     "DB_DIGIT".SM.G31_FAN01;
      U     "DB_GRP_31".FAN03.SM.MotorOn;
      U     "DB_DIGIT".SM.G31_FAN03;
      U     "DB_GRP_31".FAN31.SM.MotorOn;
      U     "DB_DIGIT".SM.G31_FAN31;
      UN    "DB_PROG_L1".OVEN.SM.SwitchOffProduction;
      =     "DB_PROG_L1".OVEN.SM.CoolingZoneON;
NETWORK
TITLE =PRODUCTION BREAK MODE
//
//********************** SET OVEN PRODUCTION BREAK MODE ************************
//
NETWORK
TITLE =OPERATION IN CASE OF CONVEYOR MALFUNCTION ON (PAP 3.1)

      U     "LOG_1";
      UN    "DB_PROG_L1".OVEN.SM.SwitchOffProduction;
      U(    ;
      O     "DB_PROG_L1".OVEN.SM.ProductionON;
      O     "DB_PROG_L1".OVEN.SM.PreHeatingON;
      )     ;
      U(    ;
      O     "DB_CONVEYORS_L1".IN.MalfunctionConveyors;
      ON    "DB_PROG_L1".OVEN.SM.ChainIsoN;
      )     ;
      L     S5T#10M;
      SE    "TPause_Malfun_Conv_L1";
      NOP   0;
      NOP   0;
      NOP   0;
      U     "TPause_Malfun_Conv_L1";
      =     "Conv_MalfunctionON_L1";
      =     "DB_PROG_L1".OVEN.SM.ConvMalfunction_ON;
NETWORK
TITLE =PRODUCTION OFF MODE
//
//************************** SET OVEN OFF MODE *****************************
//
//
      U(    ;
      O     "DB_PROG_L1".OVEN.SM.SwitchOffProduction;
      O     "DB_PROG_L1".OVEN.SM.OvenOFF;
      )     ;
      U(    ;
      O     "DB_CONVEYORS_L1".IN.MalfunctionConveyors;
      O     ;
      UN    "DB_CONVEYORS_L1".IN.MalfunctionConveyors;
      U     "DB_CONVEYORS_L1".IN.ConveyorsEmpty;
      O     "DB_PROG_L1".OVEN.SM.SwitchOnECooling;
      ON    "FDB_DIGIT".M0_FIRE_ALARM_OK;
      )     ;
      =     L      6.0;
      U     L      6.0;
      BLD   102;
      =     "OvenOFF_AfterRun_L1";
      U     L      6.0;
      L     S5T#1H;
      SE    "Timer_AfterRun_L1";
      NOP   0;
      NOP   0;
      NOP   0;
      U     "Timer_AfterRun_L1";
      =     "Timer_AfterRun_Done_L1";
      U     L      6.0;
      BLD   102;
      =     "CoolZone_OFF_L1";
NETWORK
TITLE =BURNER IS OFF, NOT IN OPERATION

      UN    "DB_GRP_21".BRN04.SM.INC_Running;
      UN    "DB_GRP_21".BRN04.SM.INC_InOperation;
      =     "Burner_IsOFF_L1";
NETWORK
TITLE =BURNER ZONE 21RIT06, TEMPERATURE OK AFTER RUN

      U     "LOG_1";
      =     L      6.0;
      U     L      6.0;
      U(    ;
      L     "DB_GRP_21".BRN04.PV.ActTemperature;
      L     300;
      <=I   ;
      )     ;
      U(    ;
      L     "DB_GRP_21".RIT06.PV.AV;
      L     1.200000e+002;
      <=R   ;
      )     ;
      =     "TempOk_BRN_AfterRun_L1";
      U     L      6.0;
      U(    ;
      L     "DB_GRP_03".CLT03.PV.AV;
      L     1.350000e+002;
      <=R   ;
      )     ;
      U(    ;
      L     "DB_GRP_04".CLT03.PV.AV;
      L     1.350000e+002;
      <=R   ;
      )     ;
      U(    ;
      L     "DB_GRP_11".CLT03.PV.AV;
      L     1.350000e+002;
      <=R   ;
      )     ;
      U(    ;
      L     "DB_GRP_12".CLT03.PV.AV;
      L     1.350000e+002;
      <=R   ;
      )     ;
      U     "TempOk_BRN_AfterRun_L1";
      =     "TempOk_Ovens_AfterRun_L1";
NETWORK
TITLE =OFF EXHAUST AIR FAN =20FAN01 AND FRESH AIR FAN =15FAN01
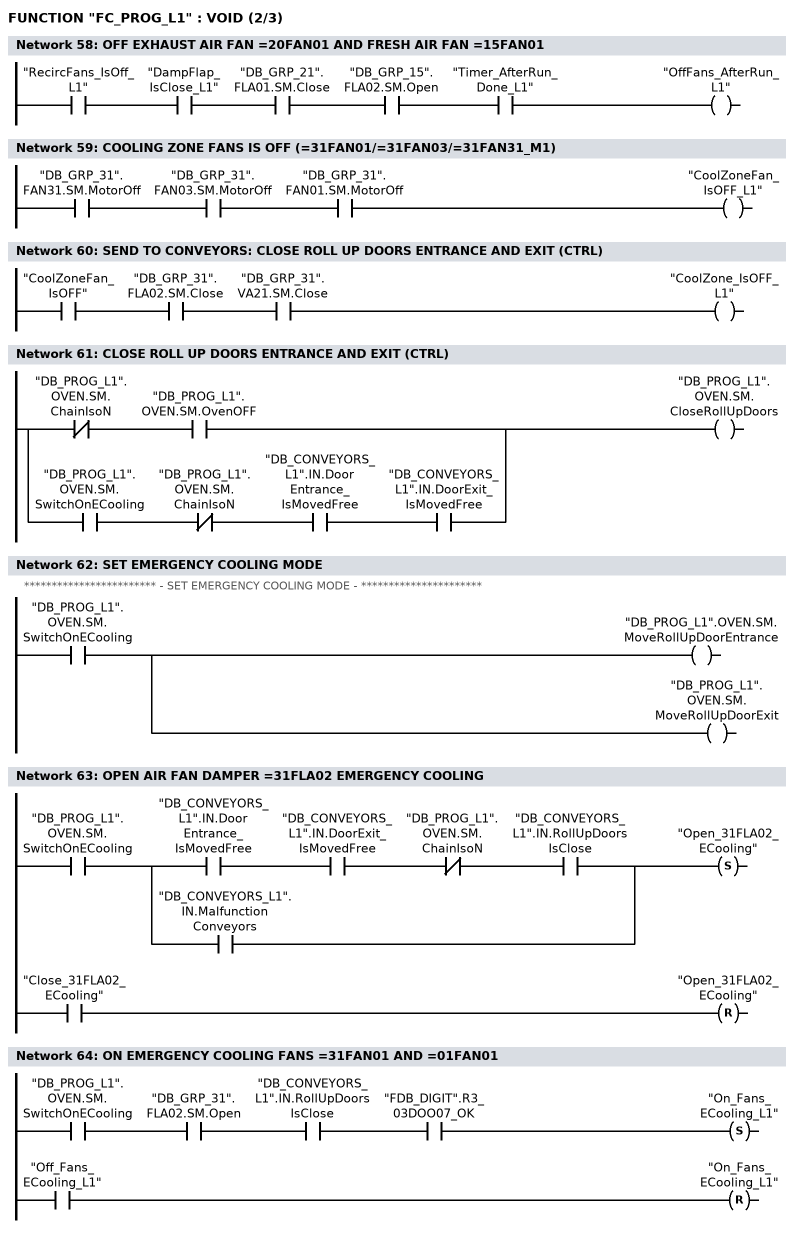
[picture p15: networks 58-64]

      U     "RecircFans_IsOff_L1";
      U     "DampFlap_IsClose_L1";
      U     "DB_GRP_21".FLA01.SM.Close;
      U     "DB_GRP_15".FLA02.SM.Open;
      U     "Timer_AfterRun_Done_L1";
      =     "OffFans_AfterRun_L1";
NETWORK
TITLE =COOLING ZONE FANS IS OFF (=31FAN01/=31FAN03/=31FAN31_M1)

      U     "DB_GRP_31".FAN31.SM.MotorOff;
      U     "DB_GRP_31".FAN03.SM.MotorOff;
      U     "DB_GRP_31".FAN01.SM.MotorOff;
      =     "CoolZoneFan_IsOFF_L1";
NETWORK
TITLE =SEND TO CONVEYORS: CLOSE ROLL UP DOORS ENTRANCE AND EXIT (CTRL)

      U     "CoolZoneFan_IsOFF";
      U     "DB_GRP_31".FLA02.SM.Close;
      U     "DB_GRP_31".VA21.SM.Close;
      =     "CoolZone_IsOFF_L1";
NETWORK
TITLE =CLOSE ROLL UP DOORS ENTRANCE AND EXIT (CTRL)

      UN    "DB_PROG_L1".OVEN.SM.ChainIsoN;
      U     "DB_PROG_L1".OVEN.SM.OvenOFF;
      O     ;
      U     "DB_PROG_L1".OVEN.SM.SwitchOnECooling;
      UN    "DB_PROG_L1".OVEN.SM.ChainIsoN;
      U     "DB_CONVEYORS_L1".IN.DoorEntrance_IsMovedFree;
      U     "DB_CONVEYORS_L1".IN.DoorExit_IsMovedFree;
      =     "DB_PROG_L1".OVEN.SM.CloseRollUpDoors;
NETWORK
TITLE =SET EMERGENCY COOLING MODE
//
//************************ - SET EMERGENCY COOLING MODE - **********************
//
      U     "DB_PROG_L1".OVEN.SM.SwitchOnECooling;
      =     "DB_PROG_L1".OVEN.SM.MoveRollUpDoorEntrance;
      =     "DB_PROG_L1".OVEN.SM.MoveRollUpDoorExit;
NETWORK
TITLE =OPEN AIR FAN DAMPER =31FLA02 EMERGENCY COOLING

      U     "DB_PROG_L1".OVEN.SM.SwitchOnECooling;
      U(    ;
      U     "DB_CONVEYORS_L1".IN.DoorEntrance_IsMovedFree;
      U     "DB_CONVEYORS_L1".IN.DoorExit_IsMovedFree;
      UN    "DB_PROG_L1".OVEN.SM.ChainIsoN;
      U     "DB_CONVEYORS_L1".IN.RollUpDoorsIsClose;
      O     "DB_CONVEYORS_L1".IN.MalfunctionConveyors;
      )     ;
      S     "Open_31FLA02_ECooling";
      U     "Close_31FLA02_ECooling";
      R     "Open_31FLA02_ECooling";
      NOP   0;
NETWORK
TITLE =ON EMERGENCY COOLING FANS =31FAN01 AND =01FAN01

      U     "DB_PROG_L1".OVEN.SM.SwitchOnECooling;
      U     "DB_GRP_31".FLA02.SM.Open;
      U     "DB_CONVEYORS_L1".IN.RollUpDoorsIsClose;
      U     "FDB_DIGIT".R3_03DOO07_OK;
      S     "On_Fans_ECooling_L1";
      U     "Off_Fans_ECooling_L1";
      R     "On_Fans_ECooling_L1";
      NOP   0;
NETWORK
TITLE =SET EMERGENCY COOLING TIME 180 MIN
//SET TIMER T_7_1_1
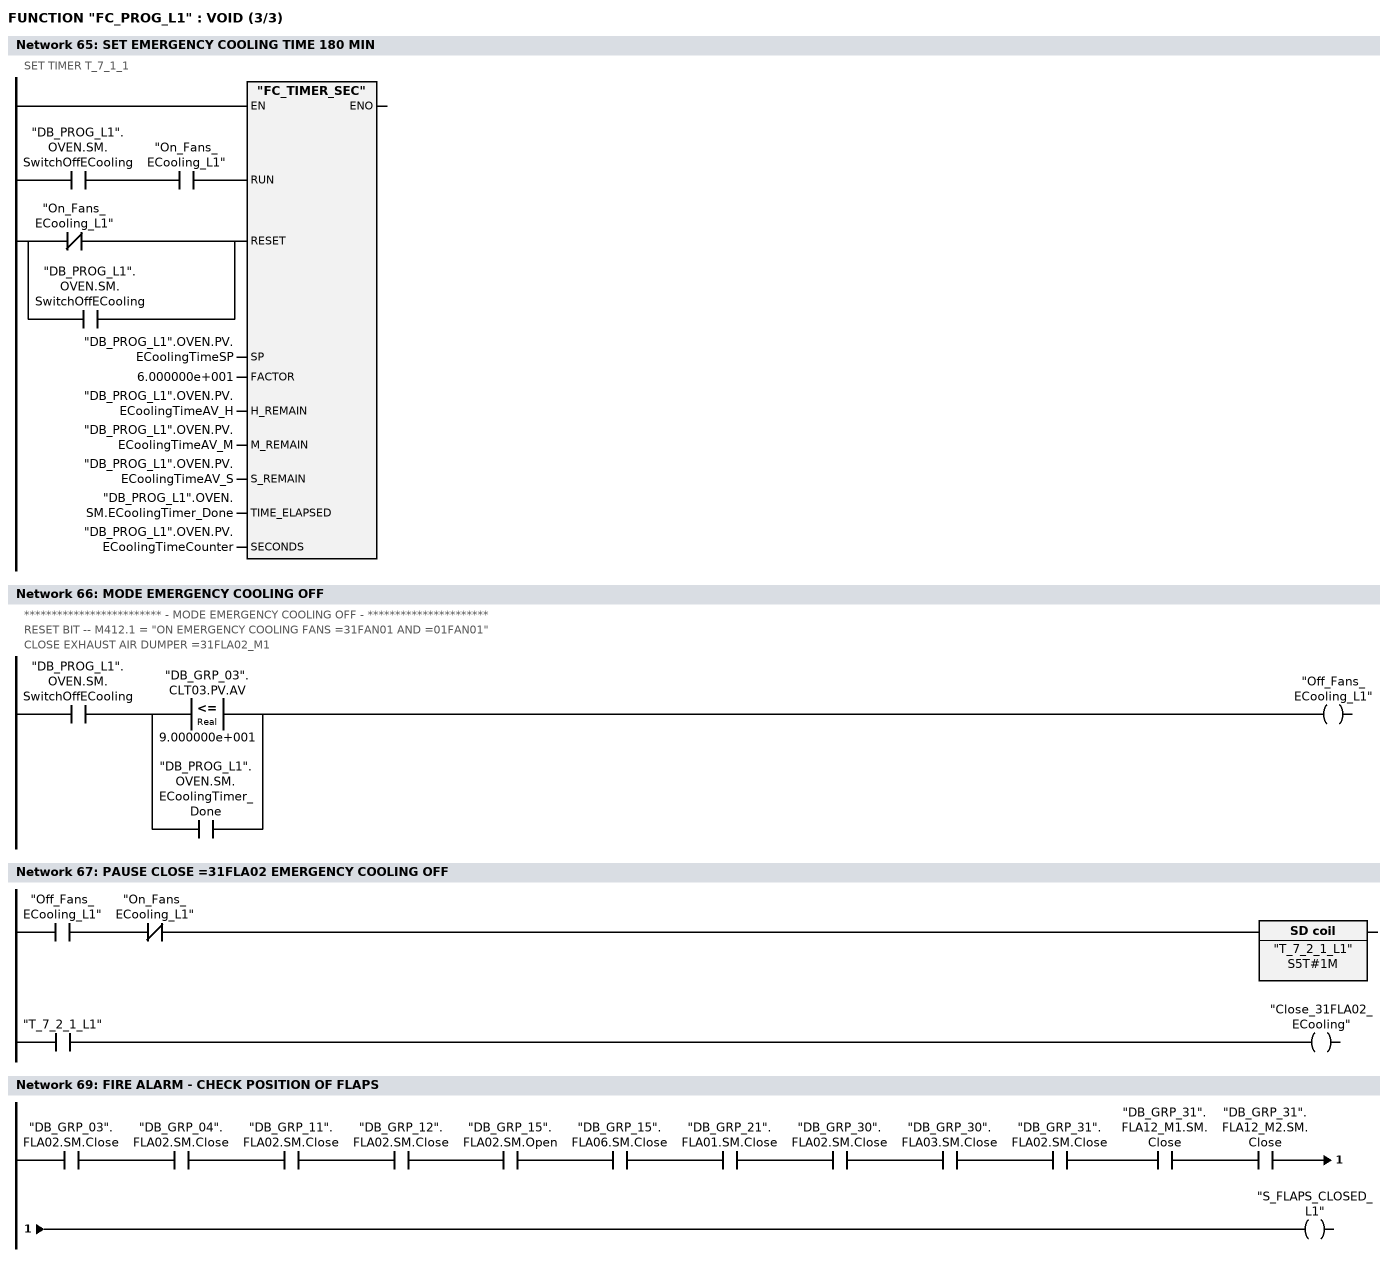
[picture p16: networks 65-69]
      U     "DB_PROG_L1".OVEN.SM.SwitchOffECooling;
      U     "On_Fans_ECooling_L1";
      =     L      6.0;
      BLD   103;
      U(    ;
      ON    "On_Fans_ECooling_L1";
      O     "DB_PROG_L1".OVEN.SM.SwitchOffECooling;
      )     ;
      =     L      6.1;
      BLD   103;
      CALL "FC_TIMER_SEC" (
           RUN                      := L      6.0,
           RESET                    := L      6.1,
           SP                       := "DB_PROG_L1".OVEN.PV.ECoolingTimeSP,
           FACTOR                   := 6.000000e+001,
           H_REMAIN                 := "DB_PROG_L1".OVEN.PV.ECoolingTimeAV_H,
           M_REMAIN                 := "DB_PROG_L1".OVEN.PV.ECoolingTimeAV_M,
           S_REMAIN                 := "DB_PROG_L1".OVEN.PV.ECoolingTimeAV_S,
           TIME_ELAPSED             := "DB_PROG_L1".OVEN.SM.ECoolingTimer_Done,
           SECONDS                  := "DB_PROG_L1".OVEN.PV.ECoolingTimeCounter);
      NOP   0;
NETWORK
TITLE =MODE EMERGENCY COOLING OFF
//
//************************* - MODE EMERGENCY COOLING OFF - **********************
//
//RESET BIT -- M412.1 = "ON EMERGENCY COOLING FANS =31FAN01 AND =01FAN01"
//CLOSE EXHAUST AIR DUMPER =31FLA02_M1
//
      U     "DB_PROG_L1".OVEN.SM.SwitchOffECooling;
      U(    ;
      O(    ;
      L     "DB_GRP_03".CLT03.PV.AV;
      L     9.000000e+001;
      <=R   ;
      )     ;
      O     "DB_PROG_L1".OVEN.SM.ECoolingTimer_Done;
      )     ;
      =     "Off_Fans_ECooling_L1";
NETWORK
TITLE =PAUSE CLOSE =31FLA02 EMERGENCY COOLING OFF

      U     "Off_Fans_ECooling_L1";
      UN    "On_Fans_ECooling_L1";
      L     S5T#1M;
      SE    "T_7_2_1_L1";
      NOP   0;
      NOP   0;
      NOP   0;
      U     "T_7_2_1_L1";
      =     "Close_31FLA02_ECooling";
NETWORK
TITLE =********** END CYCLE OF OVEN *************

NETWORK
TITLE =FIRE ALARM - CHECK POSITION OF FLAPS

      U     "DB_GRP_03".FLA02.SM.Close;
      U     "DB_GRP_04".FLA02.SM.Close;
      U     "DB_GRP_11".FLA02.SM.Close;
      U     "DB_GRP_12".FLA02.SM.Close;
      U     "DB_GRP_15".FLA02.SM.Open;
      U     "DB_GRP_15".FLA06.SM.Close;
      U     "DB_GRP_21".FLA01.SM.Close;
      U     "DB_GRP_30".FLA02.SM.Close;
      U     "DB_GRP_30".FLA03.SM.Close;
      U     "DB_GRP_31".FLA02.SM.Close;
      U     "DB_GRP_31".FLA12_M1.SM.Close;
      U     "DB_GRP_31".FLA12_M2.SM.Close;
      =     "S_FLAPS_CLOSED_L1";
NETWORK
TITLE =END

END_FUNCTION

